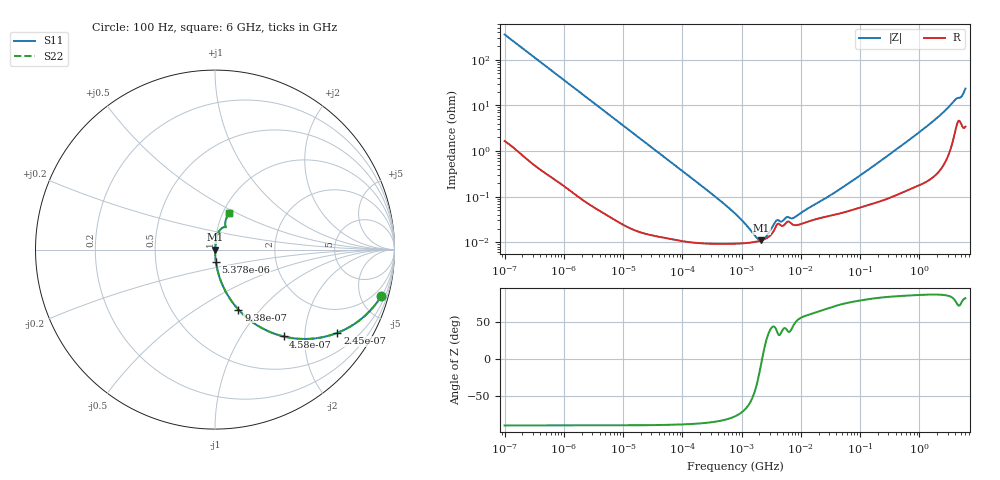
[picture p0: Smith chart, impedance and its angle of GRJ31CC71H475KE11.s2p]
!Murata Part Number: GRJ31CC71H475KE11
!These Parameters are Measured in Series Mode Connection
!Data Generated on Jun 19, 2026
!  o--ll--o
!Port1  Port2
!  o------o
!Operation Temp=25[degC], DC Bias Voltage=0[V]
!Freq. Start=100[Hz] Stop=6[GHz] 401[Steps]
# Hz S RI R 50
!Freq.(Hz) S11(Real) S11(Imag) S21(Real) S21(Imag) S12(Real) S12(Imag) S22(Real) S22(Imag)
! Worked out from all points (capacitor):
!   401 points, 100 Hz to 6 GHz, reference 50 ohm
!   read as one part in series: C = 4.43 uF near 109 Hz
!   lowest |Z| = 11.1 mohm at 2.169 MHz (marker M1)
!   series resonance near 2.226 MHz, so ESL is about 1.2 nH
!   S11 on the Smith chart (normalised r, x): 100 Hz: 1.03, -7.17; 245 Hz: 1.01, -2.94; 458 Hz: 1.01, -1.57; 938 Hz: 1.00, -0.77; 5.378 kHz: 1.00, -0.13; 6 GHz: 1.07, +0.46
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100  0.9268 -0.2582  0.0732 0.2582  0.0732 0.2582  0.9268 -0.2582
164  0.827 -0.376  0.173 0.376  0.173 0.376  0.827 -0.376
245  0.6825 -0.4633  0.3175 0.4633  0.3175 0.4633  0.6825 -0.4633
458  0.3823 -0.4838  0.6177 0.4838  0.6177 0.4838  0.3823 -0.4838
938  0.1301 -0.334  0.8699 0.334  0.8699 0.334  0.1301 -0.334
2008  0.0322 -0.1741  0.9678 0.1741  0.9678 0.1741  0.0322 -0.1741
5378  0.00491 -0.0671  0.9951 0.0671  0.9951 0.0671  0.00491 -0.0671
40335  0.000213 -0.00903  0.9998 0.00903  0.9998 0.00903  0.000213 -0.00903
774597  9.29e-05 -0.000417  0.9999 0.000417  0.9999 0.000417  9.29e-05 -0.000417
1813585  0.000104 -6.94e-05  0.9999 6.94e-05  0.9999 6.94e-05  0.000104 -6.94e-05
2169299  0.00011 -8.7e-06  0.9999 8.7e-06  0.9999 8.7e-06  0.00011 -8.7e-06
2594782  0.000121 5.37e-05  0.9999 -5.37e-05  0.9999 -5.37e-05  0.000121 5.37e-05
3882480  0.000234 0.000188  0.9998 -0.000188  0.9998 -0.000188  0.000234 0.000188
5809218  0.000276 0.000224  0.9997 -0.000224  0.9997 -0.000224  0.000276 0.000224
7599586  0.000239 0.000246  0.9998 -0.000246  0.9998 -0.000246  0.000239 0.000246
1.555665e7  0.000304 0.000546  0.9997 -0.000546  0.9997 -0.000546  0.000304 0.000546
4.983056e7  0.000442 0.00151  0.9996 -0.00151  0.9996 -0.00151  0.000442 0.00151
3.124326e8  0.001 0.00832  0.999 -0.00832  0.999 -0.00832  0.001 0.00832
2.048624e9  0.00625 0.0542  0.9937 -0.0542  0.9937 -0.0542  0.00625 0.0542
4.009986e9  0.0405 0.1209  0.9595 -0.1209  0.9595 -0.1209  0.0405 0.1209
5.016141e9  0.0578 0.1312  0.9422 -0.1312  0.9422 -0.1312  0.0578 0.1312
6e9  0.0789 0.2056  0.9211 -0.2056  0.9211 -0.2056  0.0789 0.2056
